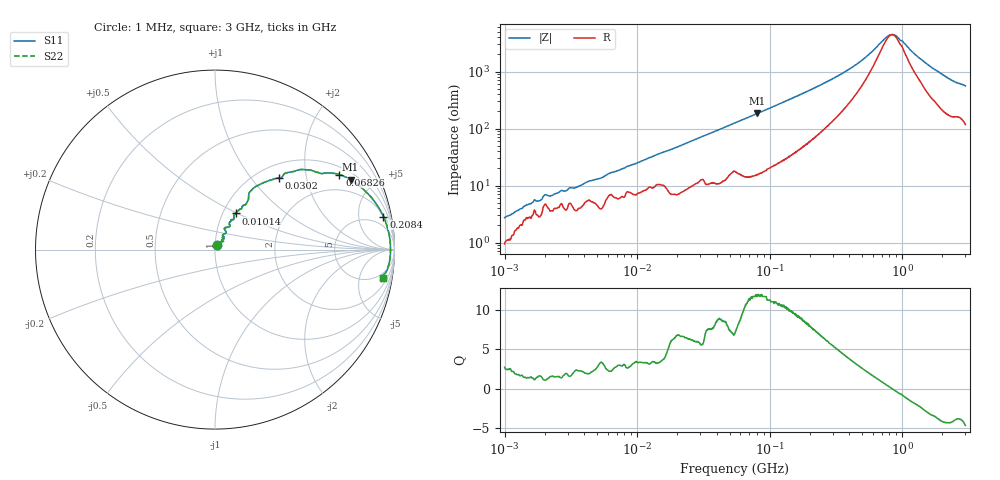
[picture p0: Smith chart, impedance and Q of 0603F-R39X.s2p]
!s-Parameter Generated by FASTRON Sdn. Bhd.
!FASTRON P/N : 0603F-R39X
!Keysight Technologies: E4991B_MY54100416_A.01.15
!Date: Thu Jun 20 13:29:47 2024
!Version  :Rev00  Thu Jun 20 13:29:47 2024
!Data & Calibration Information:
!Freq  S11  S21  S12  S22
!PortZ  Port1:50+j0  Port2:50+j0
!When reading reference impedance value at option line is always used.
! Remarks : This data is being provided solely for informational purposes.
# Hz S dB R 50
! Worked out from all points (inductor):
!   1601 points, 1 MHz to 3 GHz, reference 50 ohm
!   read as one part in series: L = 386 nH near 5.136 MHz
!   highest Q = 11.7 at 80.92 MHz (marker M1), where L = 362 nH
!   self-resonance near 840.6 MHz
!   S11 on the Smith chart (normalised r, x): 1 MHz: 1.02, +0.05; 10.14 MHz: 1.15, +0.49; 30.2 MHz: 1.25, +1.40; 68.26 MHz: 1.28, +3.11; 208.4 MHz: 2, +10; 3 GHz: 3, -11
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1000000  -31.30 68.3  -0.08 -1.5  -0.08 -1.5  -31.30 68.3
1665967  -25.50 47.0  -0.32 -2.3  -0.32 -2.3  -25.50 47.0
1850562  -25.50 55.7  -0.26 -2.6  -0.26 -2.6  -25.50 55.7
2024983  -23.60 44.1  -0.41 -2.8  -0.41 -2.8  -23.60 44.1
2249358  -23.80 54.0  -0.32 -3.1  -0.32 -3.1  -23.80 54.0
3804036  -20.20 60.5  -0.40 -5.1  -0.40 -5.1  -20.20 60.5
1.01436e7  -12.70 60.4  -0.83 -12.7  -0.83 -12.7  -12.70 60.4
1.447069e7  -10.20 55.8  -1.26 -17.2  -1.26 -17.2  -10.20 55.8
1.983357e7  -7.89 58.0  -1.33 -23.5  -1.33 -23.5  -7.89 58.0
3.019602e7  -5.42 48.1  -2.43 -31.8  -2.43 -31.8  -5.42 48.1
4.118017e7  -3.70 43.0  -3.26 -40.5  -3.26 -40.5  -3.70 43.0
5.504702e7  -2.65 35.2  -4.71 -46.9  -4.71 -46.9  -2.65 35.2
6.826239e7  -1.84 31.1  -5.70 -53.7  -5.70 -53.7  -1.84 31.1
8.092269e7  -1.41 27.3  -6.74 -57.8  -6.74 -57.8  -1.41 27.3
1.250659e8  -0.75 18.6  -9.89 -65.9  -9.89 -65.9  -0.75 18.6
2.083556e8  -0.39 11.1  -14.20 -71.5  -14.20 -71.5  -0.39 11.1
4.369573e8  -0.22 4.2  -22.30 -68.8  -22.30 -68.8  -0.22 4.2
7.925923e8  -0.19 0.4  -32.80 -15.6  -32.80 -15.6  -0.19 0.4
8.982141e8  -0.19 -0.4  -32.70 17.4  -32.70 17.4  -0.19 -0.4
1.629261e9  -0.23 -4.3  -22.00 68.5  -22.00 68.5  -0.23 -4.3
2.335937e9  -0.35 -7.5  -17.40 69.3  -17.40 69.3  -0.35 -7.5
3e9  -0.44 -9.6  -15.40 68.3  -15.40 68.3  -0.44 -9.6
